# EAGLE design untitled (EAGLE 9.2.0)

## Sheet 1 of 3: valve and pumps
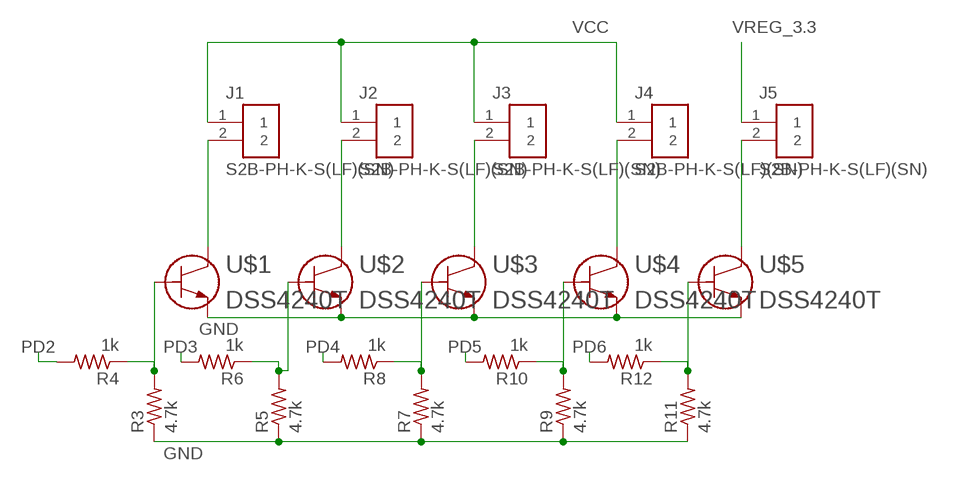
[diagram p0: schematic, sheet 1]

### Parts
J1  S2B-PH-K-S(LF)(SN)  [JST_S2B-PH-K-S(LF)(SN)]
J2  S2B-PH-K-S(LF)(SN)  [JST_S2B-PH-K-S(LF)(SN)]
J3  S2B-PH-K-S(LF)(SN)  [JST_S2B-PH-K-S(LF)(SN)]
J4  S2B-PH-K-S(LF)(SN)  [JST_S2B-PH-K-S(LF)(SN)]
J5  S2B-PH-K-S(LF)(SN)  [JST_S2B-PH-K-S(LF)(SN)]
R3  4.7k  R-US_R0603  [R0603]
R4  1k  R-US_R0603  [R0603]
R5  4.7k  R-US_R0603  [R0603]
R6  1k  R-US_R0603  [R0603]
R7  4.7k  R-US_R0603  [R0603]
R8  1k  R-US_R0603  [R0603]
R9  4.7k  R-US_R0603  [R0603]
R10  1k  R-US_R0603  [R0603]
R11  4.7k  R-US_R0603  [R0603]
R12  1k  R-US_R0603  [R0603]
U$1  DSS4240T  [TRANS_DTA113ZCAH-M]
U$2  DSS4240T  [TRANS_DTA113ZCAH-M]
U$3  DSS4240T  [TRANS_DTA113ZCAH-M]
U$4  DSS4240T  [TRANS_DTA113ZCAH-M]
U$5  DSS4240T  [TRANS_DTA113ZCAH-M]

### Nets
GND: R3.1 R5.1 R7.1 R9.1 R11.1 U$1.2 U$2.2 U$3.2 U$4.2 U$5.2 ; also sheet 2,3
N$1: J1.2 U$1.3
N$2: J2.2 U$2.3
N$3: J3.2 U$3.3
N$4: J4.2 U$4.3
N$5: J5.2 U$5.3
N$6: R3.2 R4.1 U$1.1
N$7: R5.2 R6.1 U$2.1
N$8: R7.2 R8.1 U$3.1
N$9: R9.2 R10.1 U$4.1
N$10: R11.2 R12.1 U$5.1
PD2: R4.2 ; also sheet 3
PD3: R6.2 ; also sheet 3
PD4: R8.2 ; also sheet 3
PD5: R10.2 ; also sheet 3
PD6: R12.2 ; also sheet 3
VCC: J1.1 J2.1 J3.1 J4.1 ; also sheet 3
VREG_3.3: J5.1 ; also sheet 3

## Sheet 2 of 3: power and jst outputs
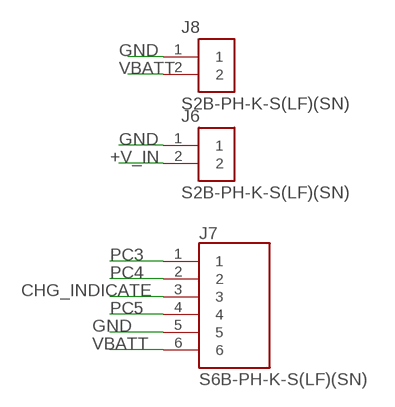
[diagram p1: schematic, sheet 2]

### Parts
J6  S2B-PH-K-S(LF)(SN)  [JST_S2B-PH-K-S(LF)(SN)]
J7  S6B-PH-K-S(LF)(SN)  [JST_S6B-PH-K-S(LF)(SN)]
J8  S2B-PH-K-S(LF)(SN)  [JST_S2B-PH-K-S(LF)(SN)]

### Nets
+V_IN: J6.2 ; also sheet 3
CHG_INDICATE: J7.3 ; also sheet 3
GND: J6.1 J7.5 J8.1 ; also sheet 1,3
PC3: J7.1 ; also sheet 3
PC4: J7.2 ; also sheet 3
PC5: J7.4 ; also sheet 3
VBATT: J7.6 J8.2 ; also sheet 3

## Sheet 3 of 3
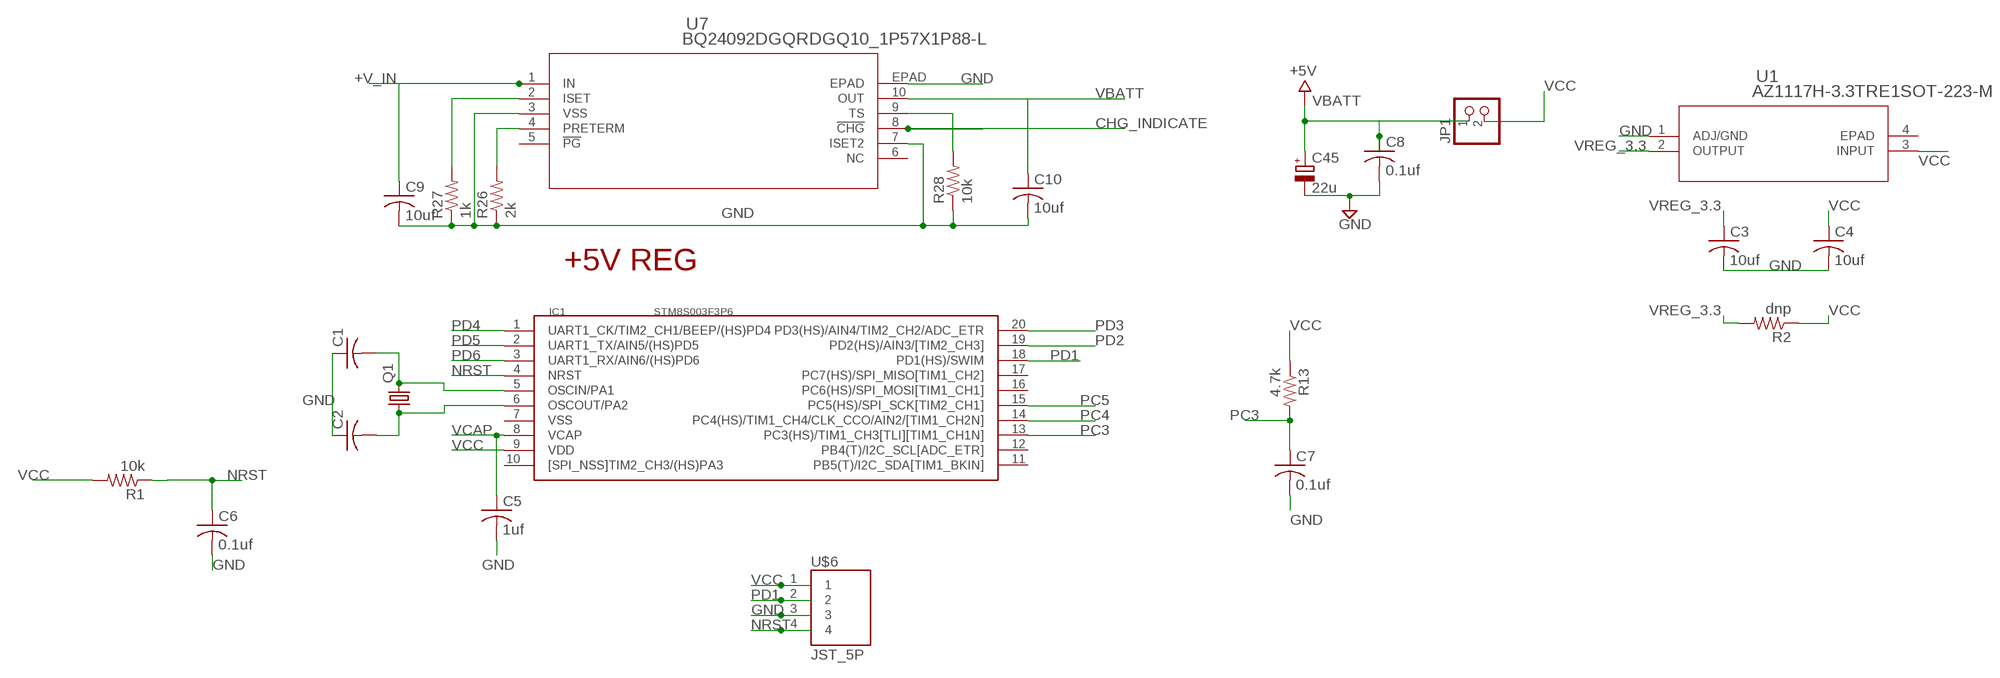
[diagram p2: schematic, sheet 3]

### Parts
C1  C-USC0805  [C0805]
C2  C-USC0805  [C0805]
C3  10uf  C-USC0805  [C0805]
C4  10uf  C-USC0805  [C0805]
C5  1uf  C-USC0805  [C0805]
C6  0.1uf  C-USC0805  [C0805]
C7  0.1uf  C-USC0805  [C0805]
C8  0.1uf  C-USC0805  [C0805]
C9  10uf  C-USC0805K  [C0805K]
C10  10uf  C-USC0805K  [C0805K]
C45  22u  CPOL-EUSMCB  [SMC_B]
IC1  STM8S003F3P6  [TSSOP20]
JP1  PINHD-1X2  [1X02]
Q1  CRYSTALHC49S  [HC49/S]
R1  10k  R-US_R0603  [R0603]
R2  dnp  R-US_R0805  [R0805]
R13  4.7k  R-US_R0603  [R0603]
R26  2k  R-US_R0603  [R0603]
R27  1k  R-US_R0603  [R0603]
R28  10k  R-US_R0603  [R0603]
U1  AZ1117H-3.3TRE1SOT-223-M  [SOT-223-M]
U7  BQ24092DGQRDGQ10_1P57X1P88-L  [DGQ10_1P57X1P88-L]
U$6  JST_5P  [JST5P]

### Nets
+V_IN: C9.1 U7.1(IN) ; also sheet 2
CHG_INDICATE: U7.8(!CHG) ; also sheet 2
GND: C1.1 C2.1 C3.2 C4.2 C5.2 C6.2 C7.2 C8.2 C9.2 C10.2 C45.- R26.1 R27.1 R28.1 U1.1(ADJ/GND) U7.3(VSS) U7.7(ISET2) U7.EPAD U$6.3 ; also sheet 1,2
N$13: C2.2 IC1.6(OSCOUT/PA2) Q1.1
N$14: C1.2 IC1.5(OSCIN/PA1) Q1.2
N$23: R27.2 U7.2(ISET)
N$24: R26.2 U7.4(PRETERM)
N$30: R28.2 U7.9(TS)
NRST: C6.1 IC1.4(NRST) R1.1 U$6.4
PC3: C7.1 IC1.13(PC3(HS)/TIM1_CH3[TLI][TIM1_CH1N]) R13.2 ; also sheet 2
PC4: IC1.14(PC4(HS)/TIM1_CH4/CLK_CCO/AIN2/[TIM1_CH2N]) ; also sheet 2
PC5: IC1.15(PC5(HS)/SPI_SCK[TIM2_CH1]) ; also sheet 2
PD1: IC1.18(PD1(HS)/SWIM) U$6.2
PD2: IC1.19(PD2(HS)/AIN3/[TIM2_CH3]) ; also sheet 1
PD3: IC1.20(PD3(HS)/AIN4/TIM2_CH2/ADC_ETR) ; also sheet 1
PD4: IC1.1(UART1_CK/TIM2_CH1/BEEP/(HS)PD4) ; also sheet 1
PD5: IC1.2(UART1_TX/AIN5/(HS)PD5) ; also sheet 1
PD6: IC1.3(UART1_RX/AIN6/(HS)PD6) ; also sheet 1
VBATT: C8.1 C10.1 C45.+ JP1.1 U7.10(OUT) ; supply symbol labelled +5V ; also sheet 2
VCAP: C5.1 IC1.8(VCAP)
VCC: C4.1 IC1.9(VDD) JP1.2 R1.2 R2.1 R13.1 U1.3(INPUT) U$6.1 ; also sheet 1
VREG_3.3: C3.1 R2.2 U1.2(OUTPUT) ; also sheet 1
Unconnected: IC1.7(VSS) IC1.10([SPI_NSS]TIM2_CH3/(HS)PA3) IC1.11(PB5(T)/I2C_SDA[TIM1_BKIN]) IC1.12(PB4(T)/I2C_SCL[ADC_ETR]) IC1.16(PC6(HS)/SPI_MOSI[TIM1_CH1]) IC1.17(PC7(HS)/SPI_MISO[TIM1_CH2]) U1.4(EPAD) U7.5(!PG) U7.6(NC)

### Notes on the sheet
- +5V REG

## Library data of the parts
C1-C10 = rcl:C-US: CAPACITOR, American symbol; SPICEPREFIX: C
C45 = rcl:CPOL-EU: POLARIZED CAPACITOR, European symbol
IC1 = STM8S003F3P6:STM8S003F3P6; AVAILABILITY: Unavailable; DESCRIPTION: STM8 STM8S Microcontroller IC 8-Bit 16MHz 8KB _8K x 8_ FLASH 20-TSSOP; MF: STMicroelectronics; MP: STM8S003F3P6; PACKAGE: TSSOP-20 STMicroelectronics; PRICE: None
J1-J6 J8 = S2B-PH-K-S_LF__SN(254):S2B-PH-K-S(LF)(SN): PH Series 2 Position 2.0 mm Through Hole Side Entry Shrouded Header; DESCRIPTION: Connector Header Through Hole, Right Angle 2 position 0.079 _2.00mm_; DIGI-KEY_PART_NUMBER: 455-1719-ND; DIGI-KEY_PURCHASE_URL: https://www.digikey.com/product-detail/en/jst-sales-america-inc/S2B-PH-K-S_LF__SN_/455-1719-ND/926626?utm_source=snapeda&utm_medium=aggregator&utm_campaign=symbol; MF: JST Sales; MP: S2B-PH-K-S_LF__SN_; PACKAGE: None
J7 = S6B-PH-K-S_LF__SN_:S6B-PH-K-S(LF)(SN): PH Series 6 Position 2 mm Pitch Through Hole Side Entry Shrouded Header; AVAILABILITY: Unavailable; DESCRIPTION: Connector Header Through Hole, Right Angle 6 position 0.079 _2.00mm_; MF: JST Sales; MP: S6B-PH-K-S_LF__SN_; PACKAGE: None; PRICE: None
JP1 = pinhead:PINHD-1X2: PIN HEADER
Q1 = crystal:CRYSTAL: CRYSTAL; OC_FARNELL: 1667008; OC_NEWARK: unknown
R1-R13 R26-R28 = rcl:R-US_: RESISTOR, American symbol; SPICEPREFIX: R
U1 = 1117reg33:AZ1117H-3.3TRE1; BUILT_BY: EMA_UL_Team; MANUFACTURER_PART_NUMBER: AZ1117H-3.3TRE1; VENDOR: Diodes Inc
U7 = bq24092dgqr:BQ24092DGQR; MANUFACTURER_PART_NUMBER: BQ24092DGQR; VENDOR: Texas Instruments
U$1-U$5 = dss4240t:DSS4240T
U$6 = jst_5p:JST_5P

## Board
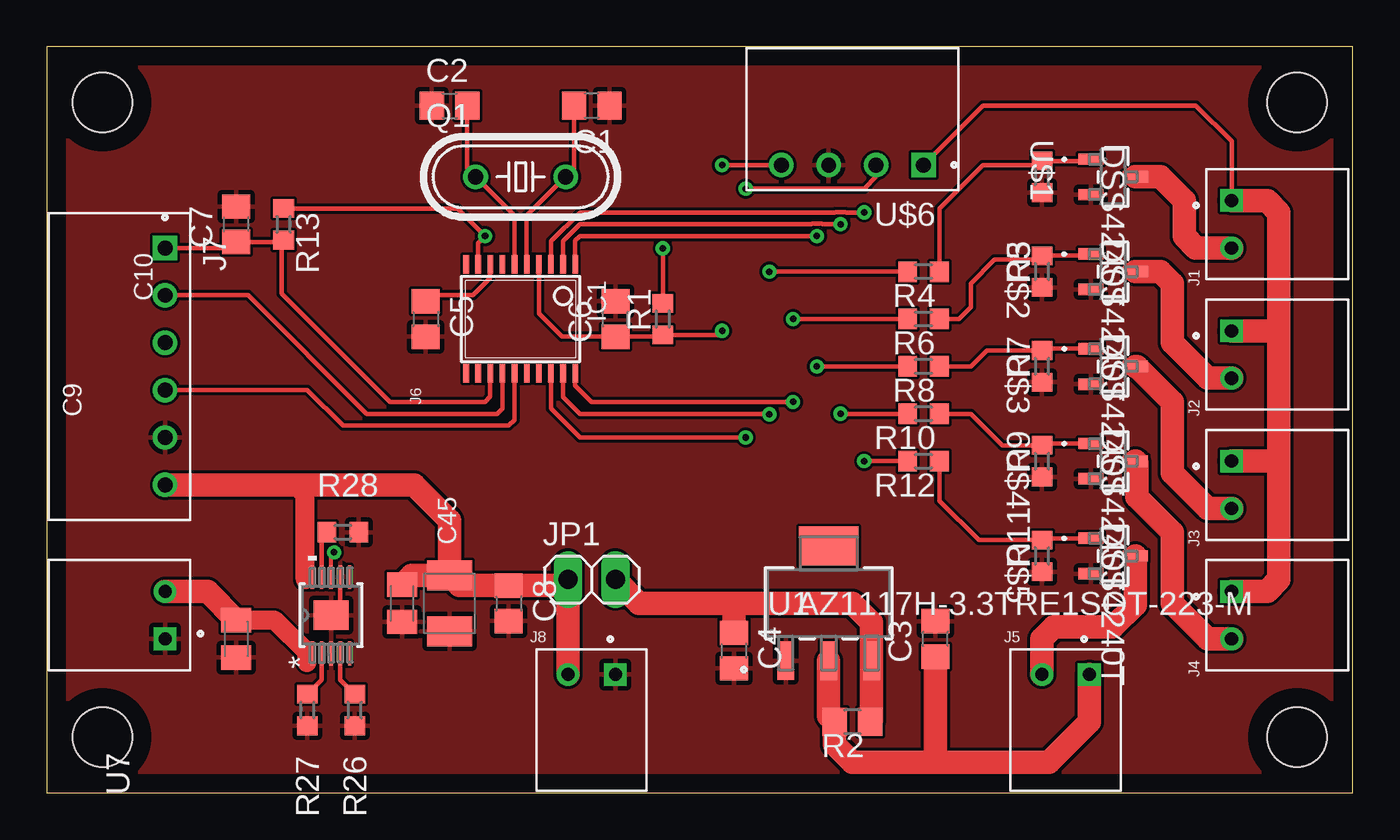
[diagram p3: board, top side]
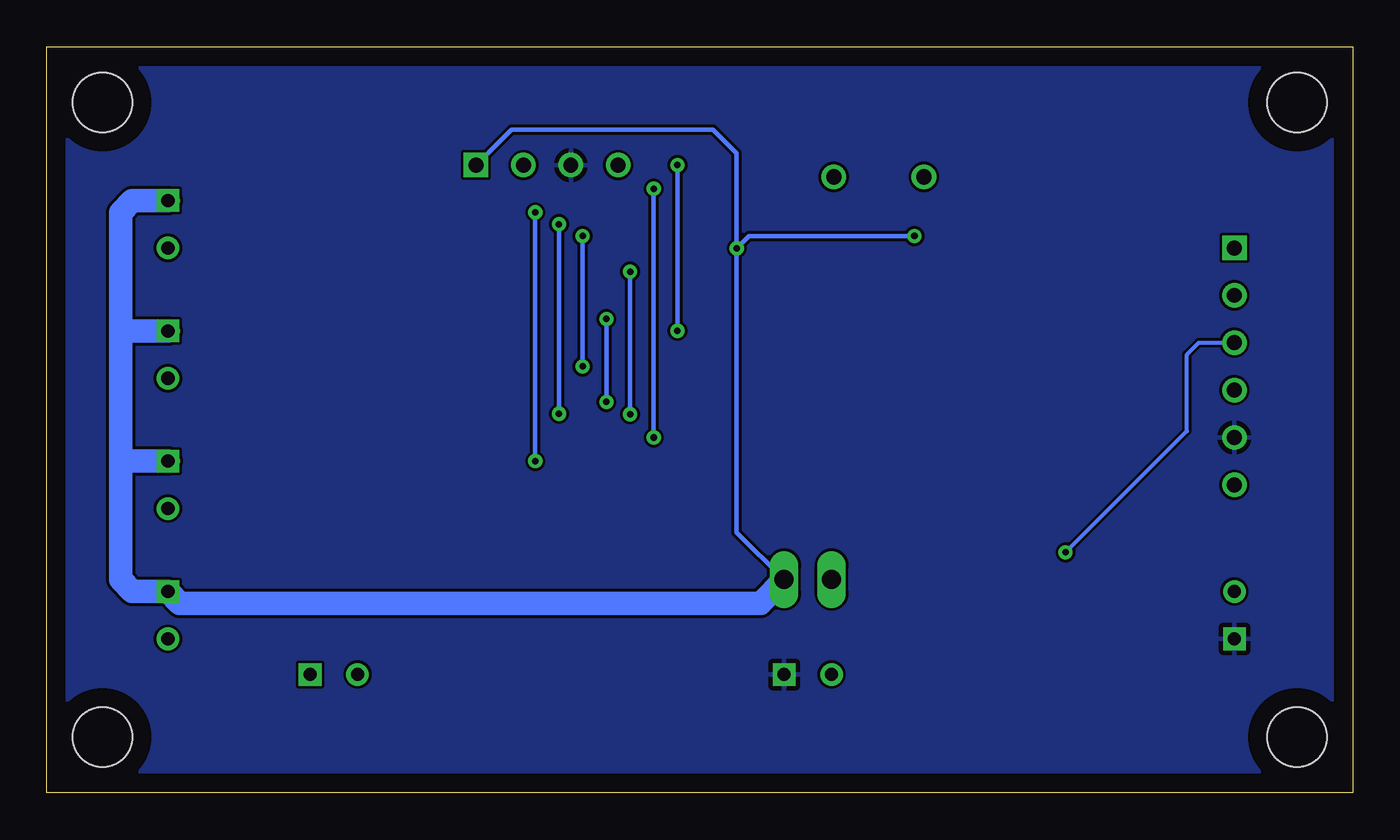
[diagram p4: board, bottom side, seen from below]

Size 70 x 40 mm. Coordinates in mm from the lower left corner, seen from the top.
Outline: 0,0 70,0 70,40 0,40 0,0
Copper layers (1*16): Top 0.035mm / dielectric 1.5mm / Bottom 0.035mm
Design rules "default": minimum track width 6mil, minimum drill 0.35mm, track to track 6mil, track to pad 6mil, pad to pad 6mil, via to via 6mil, smd to smd 6mil, copper to edge 40mil, drill to drill 6mil, minimum pad ring 10mil, minimum via ring 8mil, stop-mask expansion 4mil, vias tented up to drill 0mil, thermal gap 10mil
Holes 3.2 mm at 3,3 67,3 3,37 67,37

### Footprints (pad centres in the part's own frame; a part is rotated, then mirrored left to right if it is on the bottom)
C0805 = smd 1.3 x 1.5: 1 -0.95,0; 2 0.95,0
C0805K = smd 1.3 x 1.6: 1 -1,0; 2 1,0
SMC_B = smd 1.6 x 2.4: + -1.5,0; - 1.5,0
TSSOP20 = smd 0.305 x 0.991: 1 -2.925,-2.918; 2 -2.275,-2.918; 3 -1.625,-2.918; 4 -0.975,-2.918; 5 -0.325,-2.918; 6 0.325,-2.918; 7 0.975,-2.918; 8 1.625,-2.918; 9 2.275,-2.918; 10 2.925,-2.918; 11 2.925,2.918; 12 2.275,2.918; 13 1.625,2.918; 14 0.975,2.918; 15 0.325,2.918; 16 -0.325,2.918; 17 -0.975,2.918; 18 -1.625,2.918; 19 -2.275,2.918; 20 -2.925,2.918
JST_S2B-PH-K-S(LF)(SN) = drill 0.7 square: 1 1.27,0 | drill 0.7: 2 -1.27,0
JST_S6B-PH-K-S(LF)(SN) = drill 0.8 pad 1.2 square: 1 -6.35,0 | drill 0.8 pad 1.2: 2 -3.81,0; 3 -1.27,0; 4 1.27,0; 5 3.81,0; 6 6.35,0
1X02 = drill 1.016 long: 1 -1.27,0; 2 1.27,0
HC49/S = drill 0.813: 1 -2.413,0; 2 2.413,0
R0603 = smd 1 x 1.1: 1 -0.85,0; 2 0.85,0
R0805 = smd 1.3 x 1.5: 1 -0.95,0; 2 0.95,0
SOT-223-M = smd 0.902 x 2.066: 1 -2.3,-3.076; 2 0,-3.076; 3 2.3,-3.076 | smd 3.202 x 2.066: 4 0,3.076
DGQ10_1P57X1P88-L = smd 1.27 x 0.178: 1 -2.045,1; 2 -2.045,0.5; 3 -2.045,0; 4 -2.045,-0.5; 5 -2.045,-1; 6 2.045,-1; 7 2.045,-0.5; 8 2.045,0; 9 2.045,0.5; 10 2.045,1 | smd 1.57 x 1.88: EPAD 0,0
TRANS_DTA113ZCAH-M = smd 0.61 x 1.321: 1 -0.95,-1.194; 2 0.95,-1.194; 3 0,1.194
JST5P = drill 0.8 pad 1.2 square: 1 2.54,6.35 | drill 0.8 pad 1.2: 2 5.08,6.35; 3 7.62,6.35; 4 10.16,6.35

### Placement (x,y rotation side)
C1  29.21,36.83 180 top
C2  21.59,36.83 0 top
C3  47.62,8.26 90 top
C4  36.83,7.62 270 top
C5  20.32,25.4 270 top
C6  30.48,25.4 90 top
C7  10.16,30.48 90 top
C8  24.77,10.16 270 top
C9  10.16,8.26 270 top
C10  19.05,10.16 270 top
C45  21.59,10.16 270 top
IC1  25.4,25.4 180 top
J1  63.5,30.48 90 top
J2  63.5,23.5 90 top
J3  63.5,16.51 90 top
J4  63.5,9.53 90 top
J5  54.61,6.35 0 top
J6  6.35,9.53 270 top
J7  6.35,22.86 270 top
J8  29.21,6.35 0 top
JP1  29.21,11.43 0 top
Q1  25.4,33.02 0 top
R1  33.02,25.4 90 top
R2  43.18,3.81 180 top
R3  53.34,33.02 90 top
R4  46.99,27.94 180 top
R5  53.34,27.94 90 top
R6  46.99,25.4 180 top
R7  53.34,22.86 90 top
R8  46.99,22.86 180 top
R9  53.34,17.78 90 top
R10  46.99,20.32 180 top
R11  53.34,12.7 90 top
R12  46.99,17.78 180 top
R13  12.7,30.48 270 top
R26  16.51,4.45 90 top
R27  13.97,4.45 90 top
R28  15.88,13.97 180 top
U1  41.91,10.16 0 top
U7  15.24,9.53 90 top
U$1  57.15,33.02 270 top
U$2  57.15,27.94 270 top
U$3  57.15,22.86 270 top
U$4  57.15,17.78 270 top
U$5  57.15,12.7 270 top
U$6  49.53,40.01 180 top

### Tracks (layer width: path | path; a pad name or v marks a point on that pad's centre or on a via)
+V_IN
  Top 0.254: U7.1 14.2,7.52 13.95,7.52
  Top 1.016: C9.1 12.22,9.26 13.95,7.52 13.95,6.99
  Top 1.27: J6.2 8.62,10.79 C9.1
CHG_INDICATE  (via drill 0.35)
  Top 0.203: U7.8 15.24,12.7 15.4,12.86 v15.4,12.89
  Bottom 0.203: v15.4,12.89 8.89,19.4 8.89,23.5 8.26,24.13 J7.3
GND
  Top 0.254: U7.7 15.74,10.03 U7.EPAD
  pour Bottom: -0.64,41.27 70.48,41.27 70.48,-0.64 -0.64,-0.64
  pour Top: -0.64,40.64 71.12,40.64 71.12,-1.27 -1.27,-1.27 -1.27,40.64
N$1
  Top 1.27: J1.2 61.59,29.21 60.96,29.84 60.96,31.75 59.69,33.02 U$1.3
N$2
  Top 1.27: J2.2 62.23,22.23 60.33,24.13 60.33,27.3 59.69,27.94 U$2.3
N$3
  Top 1.27: J3.2 62.23,15.24 60.33,17.14 60.33,20.95 58.42,22.86 U$3.3
N$4
  Top 1.27: J4.2 62.23,8.26 60.33,10.16 60.33,13.97 58.42,15.88 58.42,17.7 U$4.3
N$5
  Top 1.27: U$5.3 58.34,10.08 57.15,8.89 53.98,8.89 53.34,8.26 J5.2
N$6
  Top 0.254: U$1.1 55.86,33.87 R3.2 53.12,33.66 50.16,33.66 47.84,31.33 R4.1
N$7
  Top 0.254: U$2.1 55.86,28.79 R5.2 53.12,28.57 50.8,28.57 49.53,27.3 49.53,26.04 48.9,25.4 R6.1
N$8
  Top 0.254: U$3.1 53.44,23.81 R7.2 50.38,23.71 49.53,22.86 R8.1
N$9
  Top 0.254: U$4.1 53.44,18.73 R9.2 51.22,18.63 49.53,20.32 R10.1
N$10
  Top 0.254: U$5.1 53.44,13.65 R11.2 49.95,13.55 47.84,15.66 R12.1
N$13
  Top 0.254: IC1.6 25.07,30.93 Q1.1 22.54,33.47 C2.2
N$14
  Top 0.254: IC1.5 25.73,30.93 Q1.2 28.26,33.47 C1.2
N$23
  Top 0.254: U7.2 14.74,6.07 R27.2
N$24
  Top 0.254: U7.4 15.74,6.07 R26.2
N$30
  Top 0.254: U7.9 14.74,13.62 R28.2
NRST  (via drill 0.35)
  Top 0.254: IC1.4 26.38,25.7 27.62,24.45 C6.1 32.92,24.45 R1.1 35.98,24.55 v36.2,24.77 | U$6.4 v36.2,33.66
  Bottom 0.254: v36.2,24.77 v36.2,33.66
PC3
  Top 0.254: 10.26,29.63 C7.1 | IC1.13 23.77,21.23 23.5,20.95 18.41,20.95 12.6,26.77 12.6,29.53 | C7.1 10.16,29.21 J7.1 | C7.1 12.6,29.53 | 12.6,29.53 R13.2
PC4
  Top 0.254: IC1.14 24.43,20.61 24.13,20.32 17.14,20.32 10.79,26.67 J7.2
PC5
  Top 0.254: IC1.15 25.07,20 24.77,19.68 15.88,19.68 13.97,21.59 J7.4
PD1  (via drill 0.35)
  Top 0.254: IC1.18 27.02,20.6 28.57,19.05 v37.47,19.05 | v37.47,32.38 43.81,32.38 44.45,33.02 U$6.2
  Bottom 0.254: v37.47,32.38 v37.47,19.05
PD2  (via drill 0.35)
  Top 0.254: IC1.19 27.68,21.22 28.57,20.32 38.73,20.32 v38.73,20.3 | R4.2 v38.73,27.94
  Bottom 0.254: v38.73,27.94 v38.73,20.3
PD3  (via drill 0.35)
  Top 0.254: IC1.20 28.32,21.84 29.21,20.95 v40.01,20.95 | v40.01,25.4 R6.2
  Bottom 0.254: v40.01,20.95 v40.01,25.4
PD4  (via drill 0.35)
  Top 0.254: IC1.1 28.32,29.59 28.57,29.84 40.01,29.84 40.64,29.84 v41.27,29.84 | R8.2 v41.27,22.86
  Bottom 0.254: v41.27,22.86 v41.27,29.84
PD5  (via drill 0.35)
  Top 0.254: IC1.2 27.68,29.58 28.57,30.48 40.98,30.48 41,30.5 41.55,30.5 41.57,30.48 v42.55,30.48 | v42.55,20.32 R10.2
  Bottom 0.254: v42.55,30.48 v42.55,20.32
PD6  (via drill 0.35)
  Top 0.254: IC1.3 27.02,29.57 28.57,31.11 42.25,31.11 42.27,31.14 42.82,31.14 42.84,31.11 v43.81,31.11 | R12.2 v43.81,17.78
  Bottom 0.254: v43.81,17.78 v43.81,31.11
VBATT
  Top 0.254: U7.10 14.1,11.43 13.87,11.43
  Top 1.016: 13.34,16.51 13.87,15.98 13.87,11.43
  Top 1.27: J8.2 JP1.1 27.62,11.11 C8.1 22.14,11.11 C45.+ | C45.+ 19.55,11.66 C10.1 | C45.+ 21.59,14.61 19.68,16.51 13.34,16.51 J7.6
VCAP
  Top 0.254: IC1.8 23.77,27.59 22.86,26.67 20.64,26.67 C5.1
VCC  (via drill 0.35)
  Top 0.254: IC1.9 23.12,29.48 v23.5,29.84 22.01,31.33 R13.1 | v33.02,29.19 R1.2 | J1.1 63.5,34.92 61.59,36.83 50.16,36.83 U$6.1
  Top 1.27: R2.1 44.21,3.89 U1.3 44.21,9.13 43.18,10.16 36.83,10.16 | 36.83,10.16 31.75,10.16 JP1.2 | C4.1 36.83,10.16 | J4.1 65.41,10.79 66.04,11.43 66.04,17.78 | 66.04,17.78 66.04,24.77 | 66.04,24.77 66.04,31.11 65.41,31.75 J1.1 | J2.1 66.04,24.77 | J3.1 66.04,17.78
  Bottom 0.254: v23.5,29.84 32.36,29.84 v33.02,29.19 | v33.02,29.19 33.02,34.29 34.29,35.56 45.09,35.56 U$6.1 | v33.02,29.19 33.02,13.97 JP1.2
  Bottom 1.27: JP1.2 31.75,10.16 62.87,10.16 J4.1 65.41,10.79 66.04,11.43 66.04,17.78 | 66.04,17.78 66.04,24.77 | 66.04,24.77 66.04,31.11 65.41,31.75 J1.1 | J2.1 66.04,24.77 | J3.1 66.04,17.78
VREG_3.3
  Top 1.27: U1.2 41.91,4.13 R2.2 42.23,2.6 43.18,1.65 47.62,1.65 | 47.62,1.65 53.72,1.65 55.88,3.81 J5.1 | C3.1 47.62,1.65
